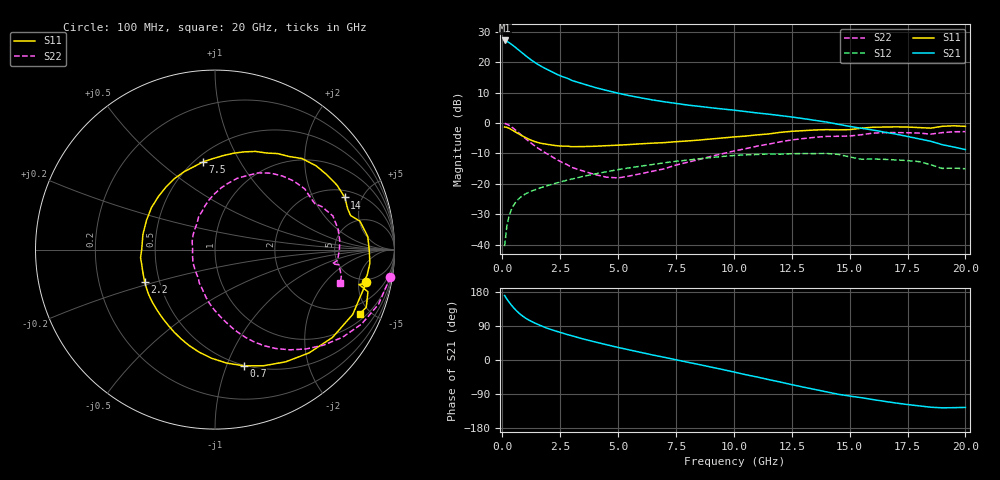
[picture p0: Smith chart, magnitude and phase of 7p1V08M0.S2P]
! Infineon Technologies  Discrete & RF Semiconductors
! bfp620
! VCE =  1.0 V,  IC =  8.0 mA
! Common Emitter S-Parameters:  Sep 2002
# GHz  S  MA  R  50
!  f  S11  S21  S12  S22
! GHz  MAG  ANG  MAG  ANG  MAG  ANG  MAG  ANG
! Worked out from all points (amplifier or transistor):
!   59 points, 100 MHz to 20 GHz, reference 50 ohm
!   highest |S21| = 27.2 dB at 100 MHz (marker M1)
!   |S21| within 3 dB of that: start of sweep to 684.3 MHz
!   unconditionally stable (mu >= 1): 4.376 GHz to 10.75 GHz; 17.02 GHz to end of sweep
!   at 1 GHz: K = 0.44, MSG = 22.8 dB, |S12| = -23.3 dB
!   at 5.5 GHz: K = 1.04, MAG = 10.6 dB, |S12| = -14.7 dB
!   at 20 GHz: K = 1.46, MAG = -0.9 dB, |S12| = -15.0 dB
!   S11 on the Smith chart (normalised r, x): 100 MHz: 4.42, -6.32; 700 MHz: 0.49, -1.15; 2.2 GHz: 0.41, -0.18; 7.5 GHz: 0.55, +0.71; 14 GHz: 2.44, +3.61; 20 GHz: 1.35, -4.35
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0.1  0.863 -12.2  22.91 170.3  0.0094 83.4  0.9886 -8.9
0.2  0.8482 -25.2  22.12 160.6  0.0206 77.5  0.9607 -18.5
0.3  0.8172 -36.8  21.02 152.0  0.0301 71.8  0.9163 -26.9
0.4  0.7787 -47.6  19.77 144.3  0.0381 66.7  0.8628 -34.4
0.5  0.739 -57.8  18.48 137.2  0.045 62.2  0.8062 -41.3
0.6  0.7014 -67.3  17.23 130.7  0.051 58.3  0.7501 -47.6
0.7  0.6667 -76.2  16.04 124.8  0.0562 55.1  0.6964 -53.3
0.8  0.6349 -84.3  14.93 119.6  0.0607 52.3  0.6462 -58.5
1  0.5786 -98.7  12.95 110.7  0.0681 48.0  0.5569 -67.2
1.3  0.5126 -116.4  10.6 100.6  0.0769 43.8  0.4506 -77.2
1.7  0.463 -135.7  8.524 89.7  0.0871 40.4  0.3533 -88.2
2.2  0.4315 -155.2  6.808 78.5  0.0995 37.5  0.2717 -100.5
3  0.4083 179.9  5.034 64.0  0.1196 32.9  0.1863 -119.5
3.5  0.4105 168.0  4.404 55.4  0.1327 29.7  0.162 -132.4
5  0.4326 136.7  3.105 33.1  0.1711 19.0  0.125 176.8
7  0.4767 104.3  2.238 7.1  0.2214 2.6  0.1768 124.6
7.5  0.4936 97.8  2.11 0.6  0.2348 -2.2  0.2034 116.8
10.5  0.6099 61.9  1.548 -38.6  0.2995 -33.9  0.3784 78.5
13.5  0.7689 27.8  1.11 -77.7  0.3147 -67.0  0.5821 41.0
14  0.7794 21.9  1.039 -84.1  0.3163 -73.5  0.6036 34.1
17  0.8662 -5.0  0.657 -113.5  0.247 -97.6  0.6969 4.2
20  0.8827 -23.8  0.366 -125.1  0.177 -110.0  0.7226 -14.8
